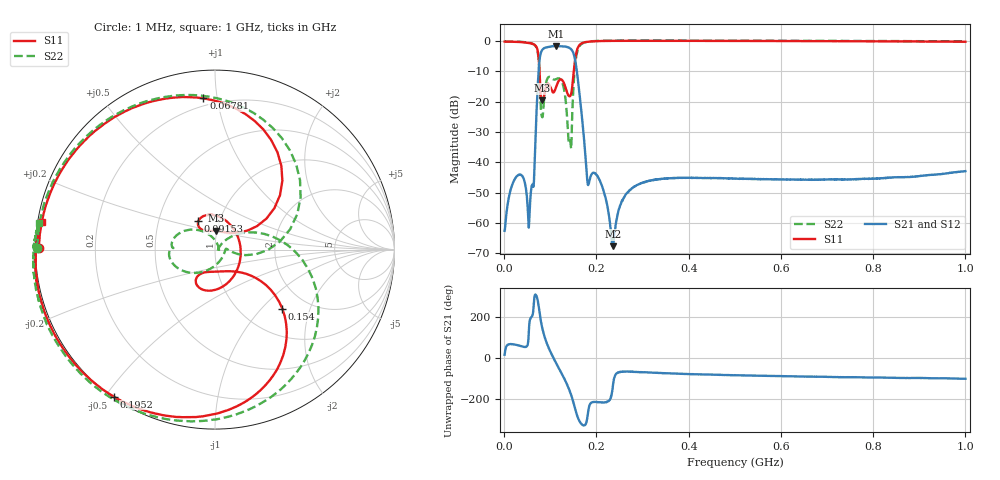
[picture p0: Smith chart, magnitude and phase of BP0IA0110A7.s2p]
!Agilent Technologies,E8358A,US41080443,A.07.50.56
!Agilent E8358A: A.07.50.56
!Date: Thursday, November 02, 2017 13:29:13
!Correction: S11(Full 2 Port(1,2))
!S21(Full 2 Port(1,2))
!S12(Full 2 Port(1,2))
!S22(Full 2 Port(1,2))
!S2P File: Measurements: S11, S21, S12, S22:
# Hz S  dB  R 50
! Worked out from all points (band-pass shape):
!   1601 points, 1 MHz to 1 GHz, reference 50 ohm
!   highest |S21| = -1.62 dB at 113.4 MHz (marker M1); lowest = -67.6 dB at 235.8 MHz (marker M2)
!   |S21| within 3 dB of the highest: 78.33 MHz to 151.5 MHz (73.19 MHz wide, 63.7 % of centre)
!   lowest |S11| = -19.6 dB at 82.17 MHz (marker M3), VSWR 1.23, Z = 49.3 + j10.5 ohm
!   |S11| at or under -10 dB: 76.71 MHz to 150.9 MHz (74.23 MHz wide, 65.2 % of centre)
!   |S22| runs from -35.5 to 0.2 dB; largest |S21 - S12| = 0.011
!   S11 on the Smith chart (normalised r, x): 1 MHz: 0.01, +0.01; 67.81 MHz: 0.15, +0.91; 91.53 MHz: 0.79, +0.26; 154 MHz: 1.51, -1.32; 195.2 MHz: 0.00, -0.53; 1 GHz: 0.01, +0.08
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1000000  -0.17 179.4  -62.54 17.1  -62.63 16.9  -0.08 179.3
2.909688e7  -0.28 159.8  -44.34 63.8  -44.36 63.8  -0.17 159.4
5.469625e7  -0.62 130.4  -58.02 170.5  -57.99 172.5  -0.57 128.0
6.780812e7  -1.46 94.4  -32.07 -49.1  -32.13 -49.0  -1.59 85.9
7.467625e7  -5.39 45.7  -10.04 -103.0  -10.10 -102.7  -6.02 23.4
8.216875e7  -19.58 87.9  -3.00 152.2  -3.06 152.3  -24.97 -7.9
9.153438e7  -14.72 120.4  -2.06 78.8  -2.11 78.9  -13.37 -146.7
1.021488e8  -15.85 56.5  -1.75 23.1  -1.81 23.0  -12.11 179.5
1.133875e8  -14.77 -56.7  -1.62 -26.9  -1.71 -27.0  -12.49 177.2
1.289969e8  -13.65 -121.0  -1.76 -92.9  -1.86 -92.9  -15.29 139.7
1.421088e8  -18.19 -86.7  -2.30 -159.3  -2.39 -159.2  -32.33 -34.4
1.539719e8  -6.04 -41.2  -6.28 112.4  -6.40 112.6  -7.74 3.0
1.677081e8  -0.76 -90.1  -23.58 39.0  -23.65 39.4  -0.97 -73.4
1.814444e8  -0.21 -112.2  -47.28 87.9  -47.36 88.1  -0.20 -103.2
1.951806e8  -0.05 -124.5  -43.44 146.6  -43.53 147.1  0.02 -118.8
2.35765e8  0.07 -143.2  -67.61 -133.1  -67.46 -134.3  0.17 -141.0
2.651106e8  0.09 -150.6  -50.32 -64.8  -50.41 -64.5  0.19 -149.2
3.344162e8  0.09 -160.8  -45.63 -71.8  -45.62 -71.2  0.20 -160.4
5.005e8  0.06 -172.4  -45.31 -82.8  -45.43 -82.8  0.15 -173.0
6.672081e8  -0.00 -179.1  -45.75 -89.7  -45.79 -89.7  0.09 -179.8
8.339162e8  -0.08 175.7  -45.03 -94.5  -45.12 -94.7  0.03 175.4
1e9  -0.20 170.9  -42.89 -100.0  -43.04 -100.3  -0.07 171.4
